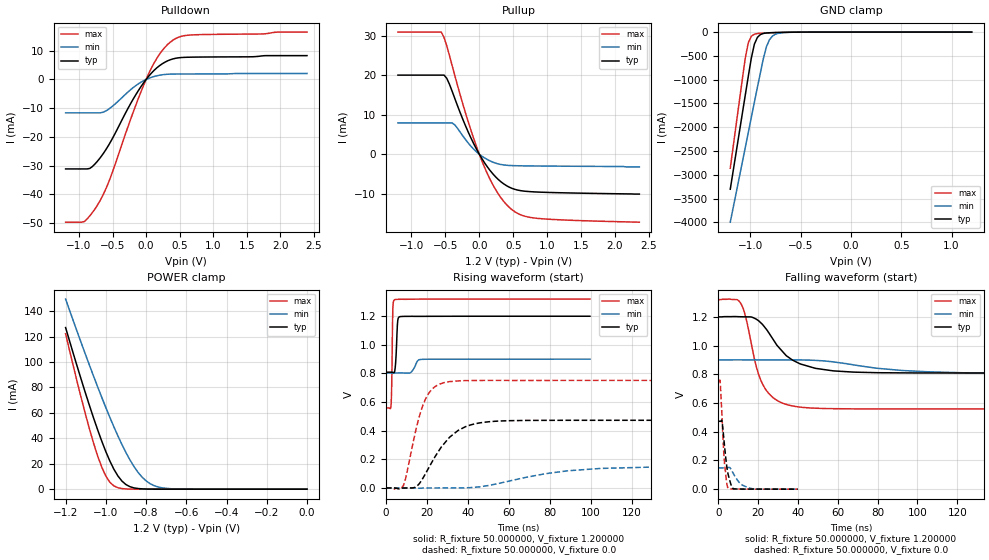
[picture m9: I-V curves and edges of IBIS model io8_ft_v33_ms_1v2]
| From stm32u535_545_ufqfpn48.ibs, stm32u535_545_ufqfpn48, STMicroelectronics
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|   Model io8_ft_v33_ms_1v2
[Model]  io8_ft_v33_ms_1v2
Model_type I/O
Polarity   Non-Inverting
Enable   Active-Low
Vinl =   0.360000V
Vinh =   0.840000V
Vmeas =  0.600000V
Cref =   50.000000pF
Rref =   100.000000M
Vref =   0.0V
C_comp   2.887200pF   2.816900pF   2.935200pF
[Temperature Range]   25.000000   0.140000k   -40.000000
[Pullup Reference]   1.200000V   0.900000V   1.320000V
[Pulldown Reference]   0.0V   0.0V   0.0V
[POWER Clamp Reference]   1.200000V   0.900000V   1.320000V
[GND Clamp Reference]   0.0V   0.0V   0.0V
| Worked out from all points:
|   slope of the pulldown table from 0 to 0.18 V, typ, clamps not added: 40.7 ohm
|   slope of the pullup table from 0 to 0.18 V, typ, clamps not added: 39.5 ohm
|   GND clamp passes 1 mA (typ) near -0.51 V on its own axis
|   POWER clamp passes 1 mA (typ) near -0.86 V on its own axis
|   rising waveform, R_fixture 50.000000, V_fixture 1.200000: 20-80 % time 745ps typ, 2.06ns min, 445ps max; typ from 0.809 V to 1.2 V
|   rising waveform, R_fixture 50.000000, V_fixture 0.0: 20-80 % time 14ns typ, 33.7ns min, 7.83ns max; typ from 0 V to 0.473 V
|   falling waveform, R_fixture 50.000000, V_fixture 1.200000: 20-80 % time 15.3ns typ, 36.8ns min, 8.75ns max; typ from 1.2 V to 0.809 V
|   falling waveform, R_fixture 50.000000, V_fixture 0.0: 20-80 % time 2.5ns typ, 4.76ns min, 1.85ns max; typ from 0.473 V to 0 V
[Pulldown]
|Voltage   I(typ)   I(min)   I(max)
-1.2V     -31.16mA   -11.61mA   -49.71mA
-920mV    -31.16mA   -11.61mA   -49.48mA
-840mV    -31mA      -11.61mA   -47.54mA
-720mV    -28.32mA   -11.61mA   -43.58mA
-560mV    -22.95mA   -10.37mA   -35.89mA
-200mV    -7.146mA   -2.964mA   -11.89mA
0V        0A         0A         0A
160mV     4.047mA    1.298mA    7.361mA
360mV     6.87mA     1.87mA     13mA
480mV     7.543mA    1.91mA     14.69mA
640mV     7.764mA    1.923mA    15.46mA
2.4V      8.316mA    2.103mA    16.52mA
[Pullup]
|Voltage   I(typ)   I(min)   I(max)
-1.2V     20.06mA    7.937mA    30.97mA
-560mV    20.06mA    7.937mA    30.97mA
-480mV    19.26mA    7.937mA    27.49mA
-360mV    14.08mA    7.422mA    19.88mA
-160mV    5.494mA    2.768mA    8.045mA
40mV      -1.16mA    -508.1uA   -1.774mA
240mV     -5.73mA    -2.256mA   -8.953mA
360mV     -7.518mA   -2.716mA   -11.96mA
480mV     -8.639mA   -2.877mA   -14.04mA
640mV     -9.31mA    -2.942mA   -15.55mA
880mV     -9.601mA   -2.986mA   -16.29mA
2.36V     -10.1mA    -3.2mA     -17.23mA
[GND_clamp]
|Voltage   I(typ)   I(min)   I(max)
-1.2V     -3.305A    -3.998A    -2.862A
-1.05V    -1.316A    -2.418A    -539.3mA
-1.02V    -921mA     -2.103A    -218.8mA
-990mV    -539.5mA   -1.788A    -87.43mA
-960mV    -252.1mA   -1.474A    -44.36mA
-930mV    -110.5mA   -1.16A     -30.32mA
-870mV    -28.03mA   -549.1mA   -21.09mA
-840mV    -18.43mA   -305.6mA   -18.27mA
-810mV    -13.9mA    -159.7mA   -15.73mA
-780mV    -11.23mA   -82.35mA   -13.37mA
-600mV    -2.976mA   -4.272mA   -3.058mA
1.2V      0A         14.74nA    0A
[POWER_clamp]
|Voltage   I(typ)   I(min)   I(max)
-1.2V     127mA      149.4mA    122.2mA
-1.12V    84.97mA    114mA      70.27mA
-1.06V    55.51mA    88.42mA    35.67mA
-1.02V    37.63mA    72.04mA    17.17mA
-1V       29.51mA    64.13mA    10.3mA
-960mV    15.69mA    48.99mA    2.571mA
-900mV    3.624mA    28.77mA    182.8uA
-840mV    490.7uA    13.24mA    11.35uA
-800mV    116.8uA    6.532mA    1.77uA
-740mV    13.2uA     1.723mA    109.1nA
-620mV    167.3nA    79.35uA    0A
0V        0A         17.84nA    0A
[Ramp]
| variable   typ   min   max
dV/dt_r  0.28373/14.02699n   88.90187m/33.65197n 0.45095/7.82166n
dV/dt_f  0.23465/15.28262n   57.88800m/36.76148n 0.45666/8.73621n
R_load = 50.000000
[Rising Waveform]
R_fixture= 50.000000
V_fixture= 1.200000
V_fixture_min= 0.900000
V_fixture_max= 1.320000
|time   V(typ)   V(min)   V(max)
0s        809mV      803.5mV    558.9mV
2.603ns   809.1mV    803.5mV    592.5mV
2.803ns   809mV      803.5mV    676.6mV
3.403ns   807.5mV    803.5mV    1.254V
4.204ns   809mV      803.5mV    1.315V
4.805ns   882.8mV    803.5mV    1.317V
5.806ns   1.169V     803.5mV    1.318V
6.807ns   1.197V     803.5mV    1.318V
17.22ns   1.199V     898.2mV    1.32V
99.7ns    1.2V       900mV      1.32V
[Rising Waveform]
R_fixture= 50.000000
V_fixture= 0.0
V_fixture_min= 0.0
V_fixture_max= 0.0
|time   V(typ)   V(min)   V(max)
0s        2.277nV    212.1nV    1.455nV
8.408ns   -560.7uV   7.063uV    11.65mV
14.41ns   5.674mV    -1.065mV   389.4mV
19.22ns   95.91mV    -413.6uV   616.5mV
24.02ns   218.5mV    -105.4uV   708.2mV
31.23ns   355.7mV    83.78uV    743.5mV
41.44ns   440.6mV    2.42mV     750.4mV
57.06ns   468.6mV    37.84mV    751.5mV
105.1ns   472.8mV    136.5mV    751.5mV
299.1ns   472.9mV    148.3mV    751.5mV
[Falling Waveform]
R_fixture= 50.000000
V_fixture= 1.200000
V_fixture_min= 0.900000
V_fixture_max= 1.320000
|time   V(typ)   V(min)   V(max)
0s        1.2V       900mV      1.32V
11.41ns   1.201V     900.6mV    1.292V
13.81ns   1.2V       900.4mV    1.198V
19.22ns   1.183V     900.5mV    847.8mV
22.22ns   1.147V     900.5mV    733.1mV
28.23ns   1.029V     900.2mV    629.8mV
37.84ns   895mV      900mV      578.1mV
49.25ns   840.6mV    896.5mV    563.7mV
80.48ns   810.9mV    841mV      559mV
299.1ns   809mV      803.5mV    558.9mV
[Falling Waveform]
R_fixture= 50.000000
V_fixture= 0.0
V_fixture_min= 0.0
V_fixture_max= 0.0
|time   V(typ)   V(min)   V(max)
0s        472.9mV    148.3mV    751.5mV
961ps     472.6mV    148.2mV    749.7mV
1.922ns   472.8mV    148.2mV    503.3mV
2.963ns   332mV      148.2mV    218.4mV
4.164ns   174mV      148mV      55.26mV
4.805ns   114.6mV    149.2mV    10.07mV
8.008ns   2.098mV    98.88mV    1.147mV
11.37ns   632.1uV    35.42mV    768.2uV
16.98ns   285.8uV    3.442mV    276.2uV
39.88ns   2.277nV    212.1nV    1.455nV
